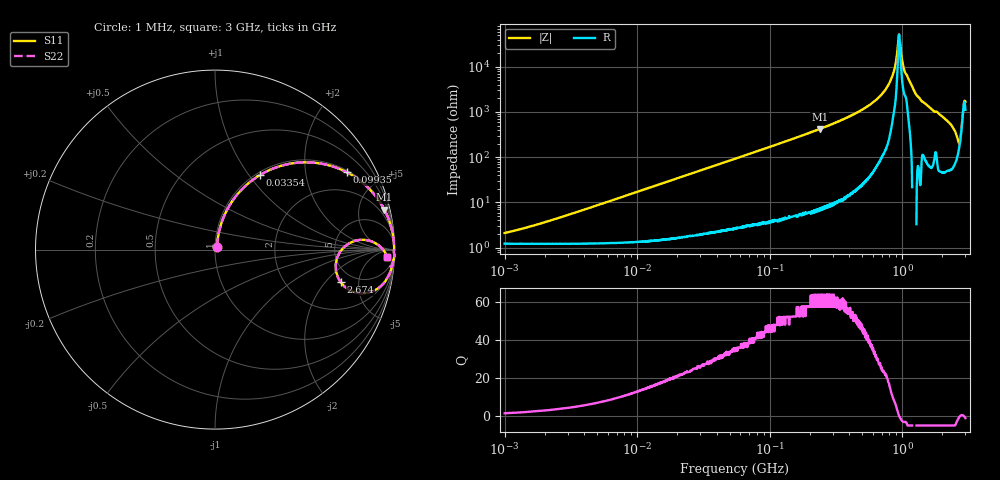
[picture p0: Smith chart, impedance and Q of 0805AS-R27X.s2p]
!s-Parameter Generated by FASTRON Sdn. Bhd.
!FASTRON P/N : 0805AS-R27X
!Keysight Technologies: E4991B_MY54100416_A.01.15
!Date: Mon Jun 15 12:53:34 2026
!Version  :Rev01  Mon Jun 15 12:53:34 2026
!Data & Calibration Information:
!Freq  S11  S21  S12  S22
!PortZ  Port1:50+j0  Port2:50+j0
!When reading reference impedance value at option line is always used.
! Remarks : This data is being provided solely for informational purposes.
# Hz S dB R 50
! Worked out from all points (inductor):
!   1601 points, 1 MHz to 3 GHz, reference 50 ohm
!   read as one part in series: L = 273 nH near 2.14 MHz
!   highest Q = 63.5 at 238.5 MHz (marker M1), where L = 282 nH
!   self-resonance near 944.3 MHz
!   S11 on the Smith chart (normalised r, x): 1 MHz: 1.02, +0.03; 33.54 MHz: 1.04, +1.14; 99.35 MHz: 1.08, +3.36; 2.674 GHz: 3.87, -2.98; 3 GHz: 23, -25
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1000000  -33.60 53.5  -0.11 -1.0  -0.11 -1.0  -33.60 53.5
3804036  -23.70 75.6  -0.12 -3.7  -0.12 -3.7  -23.70 75.6
1.447069e7  -12.50 72.9  -0.38 -13.7  -0.38 -13.7  -12.50 72.9
3.354185e7  -6.25 58.8  -1.35 -29.1  -1.35 -29.1  -6.25 58.8
5.504702e7  -3.46 46.2  -2.83 -42.2  -2.83 -42.2  -3.46 46.2
9.935083e7  -1.40 30.4  -5.90 -58.3  -5.90 -58.3  -1.40 30.4
2.083556e8  -0.36 15.3  -11.60 -73.7  -11.60 -73.7  -0.36 15.3
2.384963e8  -0.27 13.3  -12.80 -75.7  -12.80 -75.7  -0.27 13.3
5.284703e8  -0.04 4.6  -22.00 -84.1  -22.00 -84.1  -0.04 4.6
6.753166e8  -0.02 2.6  -26.80 -85.3  -26.80 -85.3  -0.02 2.6
7.925923e8  -0.01 1.4  -32.30 -85.3  -32.30 -85.3  -0.01 1.4
8.629671e8  -0.01 0.7  -37.70 -82.5  -37.70 -82.5  -0.01 0.7
9.255909e8  -0.01 0.2  -48.60 -64.6  -48.60 -64.6  -0.01 0.2
9.538021e8  -0.02 -0.0  -53.50 18.0  -53.50 18.0  -0.02 -0.0
1.048936e9  -0.04 -0.7  -37.60 71.6  -37.60 71.6  -0.04 -0.7
1.274982e9  -0.00 -2.4  -27.70 88.0  -27.70 88.0  -0.00 -2.4
2.301132e9  -0.28 -10.1  -15.10 74.5  -15.10 74.5  -0.28 -10.1
2.556106e9  -0.98 -15.4  -11.20 59.7  -11.20 59.7  -0.98 -15.4
2.673854e9  -2.80 -14.6  -9.11 31.4  -9.11 31.4  -2.80 -14.6
2.741597e9  -3.13 -0.9  -10.40 2.1  -10.40 2.1  -3.13 -0.9
2.825159e9  -1.34 3.4  -16.30 -19.3  -16.30 -19.3  -1.34 3.4
3e9  -0.34 -2.4  -24.90 46.1  -24.90 46.1  -0.34 -2.4
